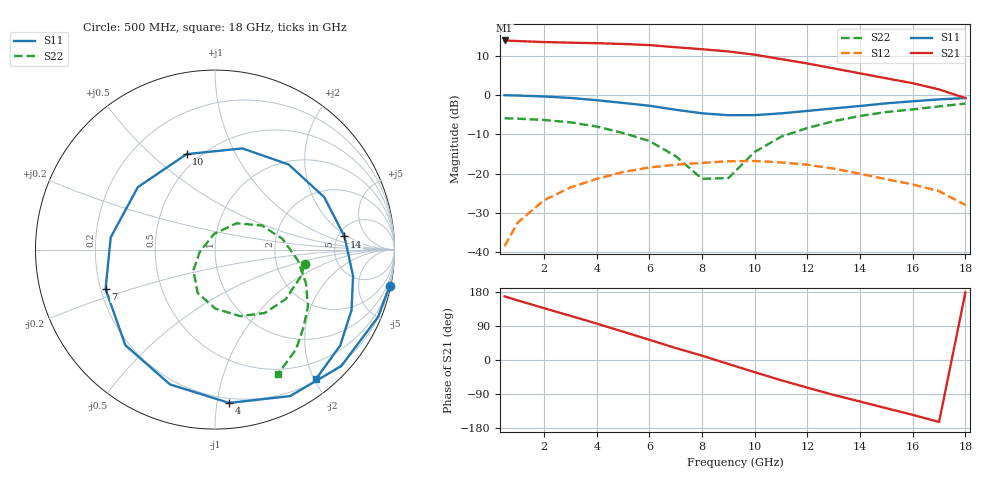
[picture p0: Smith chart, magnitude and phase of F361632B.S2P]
!ATF-36163
!2V 15mA
! last updated 11-10-95
# ghz s ma r 50
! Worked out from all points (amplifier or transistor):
!   19 points, 500 MHz to 18 GHz, reference 50 ohm
!   highest |S21| = 13.9 dB at 500 MHz (marker M1)
!   |S21| within 3 dB of that: start of sweep to 9.247 GHz
!   unconditionally stable (mu >= 1): 10.53 GHz to end of sweep
!   at 3 GHz: K = 0.35, MSG = 18.4 dB, |S12| = -23.5 dB
!   at 9 GHz: K = 0.90, MSG = 13.9 dB, |S12| = -16.8 dB
!   at 18 GHz: K = 1.49, MAG = 9.5 dB, |S12| = -28.0 dB
!   lowest NFmin = 0.48 dB at 2 GHz
!   S11 on the Smith chart (normalised r, x): 500 MHz: 0.29, -9.83; 4 GHz: 0.17, -1.08; 7 GHz: 0.22, -0.17; 10 GHz: 0.43, +0.65; 14 GHz: 5.71, +1.77; 18 GHz: 0.23, -2.03
0.5  0.994 -11.6  4.927 167.8  0.012 79.3  0.506 -9.2
1  0.983 -22.4  4.84 157.2  0.024 71.4  0.5 -18.0
2  0.957 -42.7  4.703 136.7  0.046 55.8  0.481 -35.1
3  0.917 -62.9  4.618 116.5  0.067 40.3  0.449 -51.8
4  0.858 -84.7  4.55 96.0  0.086 23.8  0.397 -69.2
5  0.792 -108.5  4.445 74.8  0.105 6.6  0.329 -89.6
6  0.73 -133.2  4.299 53.3  0.12 -10.4  0.26 -111.8
7  0.648 -160.2  4.042 31.5  0.13 -28.2  0.167 -136.1
8  0.585 173.3  3.813 11.4  0.137 -41.6  0.086 -171.3
9  0.553 141.0  3.571 -10.5  0.144 -56.7  0.088 92.9
10  0.555 106.6  3.247 -32.2  0.145 -72.0  0.189 50.9
11  0.584 74.9  2.855 -53.4  0.139 -86.8  0.295 27.1
12  0.627 49.1  2.512 -73.0  0.13 -99.5  0.381 8.9
13  0.675 25.7  2.174 -92.2  0.116 -112.0  0.465 -7.3
14  0.725 5.8  1.882 -109.6  0.1 -120.8  0.541 -20.4
15  0.783 -10.8  1.626 -127.3  0.085 -129.3  0.607 -31.5
16  0.832 -23.9  1.411 -144.7  0.073 -134.7  0.656 -41.3
17  0.879 -37.5  1.177 -163.6  0.06 -142.8  0.716 -50.9
18  0.914 -51.9  0.913 178.2  0.04 -148.8  0.778 -63.3
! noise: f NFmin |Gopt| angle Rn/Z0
2  0.48  0.834  27.73  0.372
3  0.52  0.744  41.33  0.308
5  0.61  0.602  70.9  0.191
7  0.7  0.463  103.7  0.113
9  0.82  0.307  136.4  0.075
10  0.88  0.207  168.3  0.073
12  1.03  0.182  -85.06  0.132
14  1.23  0.359  -13.13  0.315
16  1.49  0.576  20.25  0.597
18  1.86  0.696  51.32  1.103
